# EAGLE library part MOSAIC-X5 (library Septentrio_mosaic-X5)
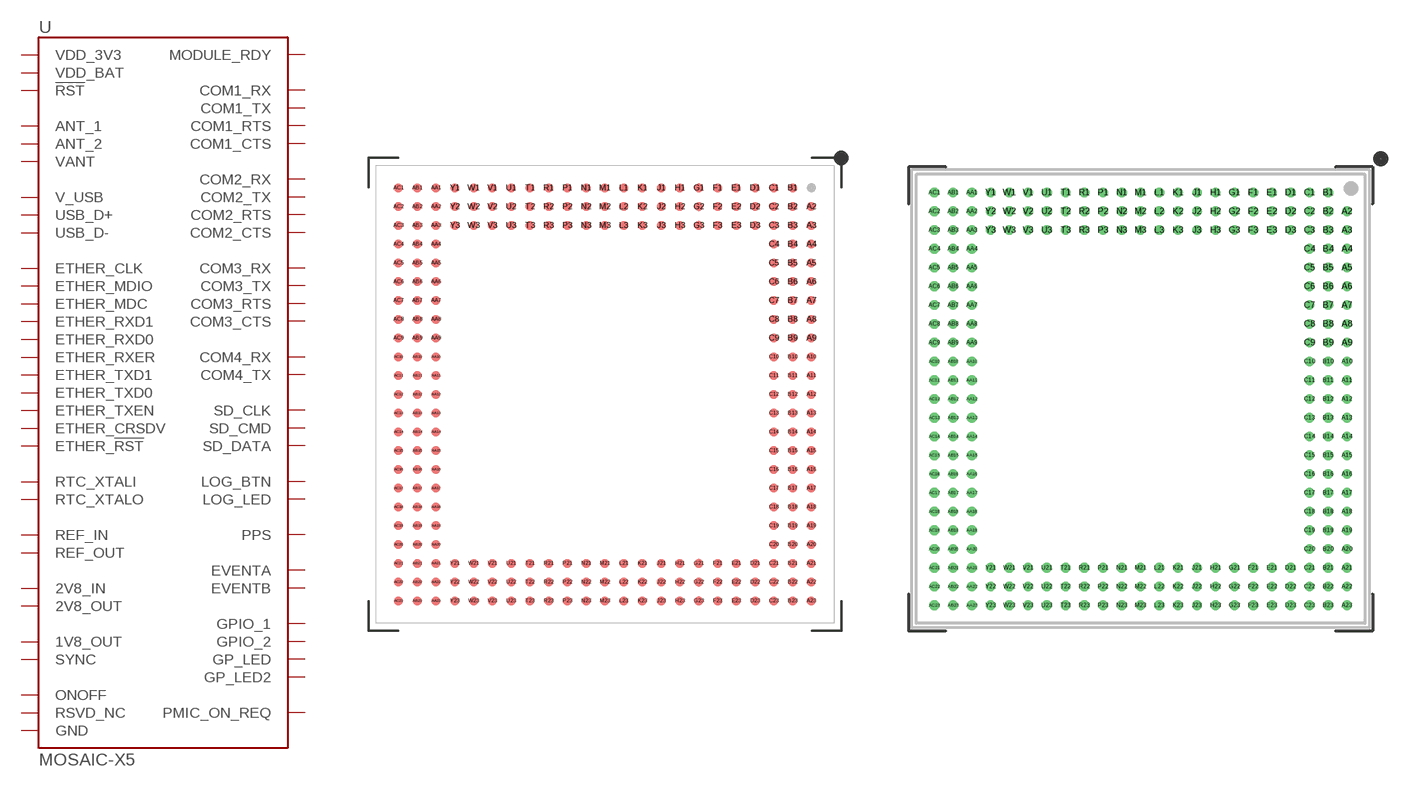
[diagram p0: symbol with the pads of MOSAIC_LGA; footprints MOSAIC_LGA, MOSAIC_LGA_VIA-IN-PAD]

Designator prefix -

## MOSAIC-X5X5 (PROD_ID: GPS-19395)  [MOSAIC_LGA]
A2  RTC_XTALO  out
A3  RTC_XTALI  in
A4  GND  pwr
A5  USB_D+
A6  USB_D-
A7  GND  pwr
A8  V_USB  in
A9  RSVD_NC  nc
A10  ONOFF  in
A11  !RST!  in
A12  MODULE_RDY  out
A13  RSVD_NC  nc
A14  GP_LED  out
A15  GND  pwr
A16  GND  pwr
A17  GND  pwr
A18  VDD_3V3  in
A19  VDD_3V3  in
A20  VDD_3V3  in
A21  GND  pwr
A22  GND  pwr
A23  GND  pwr
AA1  SD_CLK  out
AA2  ETHER_CLK  out
AA3  RSVD_NC  nc
AA4  GPIO_1  out
AA5  RSVD_NC  nc
AA6  RSVD_NC  nc
AA7  RSVD_NC  nc
AA8  RSVD_NC  nc
AA9  RSVD_NC  nc
AA10  RSVD_NC  nc
AA11  RSVD_NC  nc
AA12  RSVD_NC  nc
AA13  GND  pwr
AA14  GND  pwr
AA15  GND  pwr
AA16  GND  pwr
AA17  GND  pwr
AA18  GND  pwr
AA19  GND  pwr
AA20  GND  pwr
AA21  GND  pwr
AA22  GND  pwr
AA23  GND  pwr
AB1  SD_CMD  out
AB2  GND  pwr
AB3  GND  pwr
AB4  GND  pwr
AB5  GND  pwr
AB6  GND  pwr
AB7  GND  pwr
AB8  GND  pwr
AB9  RSVD_NC  nc
AB10  RSVD_NC  nc
AB11  RSVD_NC  nc
AB12  RSVD_NC  nc
AB13  GND  pwr
AB14  GND  pwr
AB15  GND  pwr
AB16  GND  pwr
AB17  GND  pwr
AB18  GND  pwr
AB19  GND  pwr
AB20  GND  pwr
AB21  GND  pwr
AB22  GND  pwr
AB23  GND  pwr
AC1  RSVD_NC  nc
AC2  RSVD_NC  nc
AC3  SYNC  in
AC4  1V8_OUT  out
AC5  RSVD_NC  nc
AC6  EVENTA  in
AC7  EVENTB  in
AC8  PPS  out
AC9  RSVD_NC  nc
AC10  RSVD_NC  nc
AC11  RSVD_NC  nc
AC12  RSVD_NC  nc
AC13  GND  pwr
AC14  RSVD_NC  nc
AC15  GND  pwr
AC16  REF_OUT  out
AC17  REF_IN  in
AC18  GND  pwr
AC19  GND  pwr
AC20  ANT_1  in
AC21  GND  pwr
AC22  GND  pwr
AC23  GND  pwr
B1  COM1_RX  in
B2  LOG_LED  out
B3  RSVD_NC  nc
B4  GND  pwr
B5  GND  pwr
B6  GND  pwr
B7  GND  pwr
B8  VDD_BAT  in
B9  RSVD_NC  nc
B10  RSVD_NC  nc
B11  RSVD_NC  nc
B12  RSVD_NC  nc
B13  GND  pwr
B14  RSVD_NC  nc
B15  RSVD_NC  nc
B16  PMIC_ON_REQ  out
B17  GND  pwr
B18  VDD_3V3  in
B19  VDD_3V3  in
B20  VDD_3V3  in
B21  GND  pwr
B22  RSVD_NC  nc
B23  RSVD_NC  nc
C1  COM1_RTS  out
C2  RSVD_NC  nc
C3  RSVD_NC  nc
C4  GND  pwr
C5  RSVD_NC  nc
C6  RSVD_NC  nc
C7  GND  pwr
C8  RSVD_NC  nc
C9  RSVD_NC  nc
C10  RSVD_NC  nc
C11  RSVD_NC  nc
C12  RSVD_NC  nc
C13  RSVD_NC  nc
C14  RSVD_NC  nc
C15  GND  pwr
C16  GND  pwr
C17  GND  pwr
C18  VDD_3V3  in
C19  VDD_3V3  in
C20  VDD_3V3  in
C21  RSVD_NC  nc
C22  RSVD_NC  nc
C23  GND  pwr
D1  COM1_TX  out
D2  GND  pwr
D3  COM4_RX  in
D21  GND  pwr
D22  GND  pwr
D23  GND  pwr
E1  COM1_CTS  in
E2  GND  pwr
E3  COM4_TX  out
E21  GND  pwr
E22  GND  pwr
E23  GND  pwr
F1  COM2_RX  in
F2  ETHER_!RST!  in
F3  RSVD_NC  nc
F21  GND  pwr
F22  GND  pwr
F23  GND  pwr
G1  COM2_RTS  out
G2  GND  pwr
G3  RSVD_NC  nc
G21  GND  pwr
G22  RSVD_NC  nc
G23  GND  pwr
H1  COM2_TX  out
H2  ETHER_TXD1  out
H3  RSVD_NC  nc
H21  GND  pwr
H22  GND  pwr
H23  GND  pwr
J1  COM2_CTS  in
J2  ETHER_TXD0  out
J3  RSVD_NC  nc
J21  GND  pwr
J22  GND  pwr
J23  GND  pwr
K1  COM3_RX  in
K2  GND  pwr
K3  LOG_BTN  in
K21  GND  pwr
K22  GND  pwr
K23  GND  pwr
L1  COM3_RTS  out
L2  ETHER_TXEN  out
L3  GPIO_2  out
L21  GND  pwr
L22  GND  pwr
L23  GND  pwr
M1  COM3_TX  out
M2  ETHER_RXER  in
M3  GP_LED2  out
M21  GND  pwr
M22  GND  pwr
M23  2V8_IN  in
N1  COM3_CTS  in
N2  ETHER_CRSDV  in
N3  RSVD_NC  nc
N21  GND  pwr
N22  GND  pwr
N23  2V8_OUT  out
P1  GND  pwr
P2  GND  pwr
P3  GND  pwr
P21  GND  pwr
P22  GND  pwr
P23  VANT  in
R1  RSVD_NC  nc
R2  ETHER_RXD0  in
R3  GND  pwr
R21  GND  pwr
R22  GND  pwr
R23  VANT  in
T1  RSVD_NC  nc
T2  ETHER_RXD1  in
T3  RSVD_NC  nc
T21  GND  pwr
T22  GND  pwr
T23  GND  pwr
U1  RSVD_NC  nc
U2  GND  pwr
U3  RSVD_NC  nc
U21  GND  pwr
U22  GND  pwr
U23  GND  pwr
V1  RSVD_NC  nc
V2  ETHER_MDC  out
V3  RSVD_NC  nc
V21  GND  pwr
V22  GND  pwr
V23  ANT_2  in
W1  RSVD_NC  nc
W2  ETHER_MDIO
W3  RSVD_NC  nc
W21  GND  pwr
W22  GND  pwr
W23  GND  pwr
Y1  SD_DATA
Y2  GND  pwr
Y3  RSVD_NC  nc
Y21  GND  pwr
Y22  GND  pwr
Y23  GND  pwr

## MOSAIC-X5X5_VIA-IN-PAD  [MOSAIC_LGA_VIA-IN-PAD]
Pads as for MOSAIC_LGA

## Footprint MOSAIC_LGA (pad centres in mm)
MOSAIC LGA - SMD
smd 0.6 x 0.6: A2 13.97,12.7; A3 13.97,11.43; A4 13.97,10.16; A5 13.97,8.89; A6 13.97,7.62; A7 13.97,6.35; A8 13.97,5.08; A9 13.97,3.81; A10 13.97,2.54; A11 13.97,1.27; A12 13.97,0; A13 13.97,-1.27; A14 13.97,-2.54; A15 13.97,-3.81; A16 13.97,-5.08; A17 13.97,-6.35; A18 13.97,-7.62; A19 13.97,-8.89; A20 13.97,-10.16; A21 13.97,-11.43; A22 13.97,-12.7; A23 13.97,-13.97; AA1 -11.43,13.97; AA2 -11.43,12.7; AA3 -11.43,11.43; AA4 -11.43,10.16; AA5 -11.43,8.89; AA6 -11.43,7.62; AA7 -11.43,6.35; AA8 -11.43,5.08; AA9 -11.43,3.81; AA10 -11.43,2.54; AA11 -11.43,1.27; AA12 -11.43,0; AA13 -11.43,-1.27; AA14 -11.43,-2.54; AA15 -11.43,-3.81; AA16 -11.43,-5.08; AA17 -11.43,-6.35; AA18 -11.43,-7.62; AA19 -11.43,-8.89; AA20 -11.43,-10.16; AA21 -11.43,-11.43; AA22 -11.43,-12.7; AA23 -11.43,-13.97; AB1 -12.7,13.97; AB2 -12.7,12.7; AB3 -12.7,11.43; AB4 -12.7,10.16; AB5 -12.7,8.89; AB6 -12.7,7.62; AB7 -12.7,6.35; AB8 -12.7,5.08; AB9 -12.7,3.81; AB10 -12.7,2.54; AB11 -12.7,1.27; AB12 -12.7,0; AB13 -12.7,-1.27; AB14 -12.7,-2.54; AB15 -12.7,-3.81; AB16 -12.7,-5.08; AB17 -12.7,-6.35; AB18 -12.7,-7.62; AB19 -12.7,-8.89; AB20 -12.7,-10.16; AB21 -12.7,-11.43; AB22 -12.7,-12.7; AB23 -12.7,-13.97; AC1 -13.97,13.97; AC2 -13.97,12.7; AC3 -13.97,11.43; AC4 -13.97,10.16; AC5 -13.97,8.89; AC6 -13.97,7.62; AC7 -13.97,6.35; AC8 -13.97,5.08; AC9 -13.97,3.81; AC10 -13.97,2.54; AC11 -13.97,1.27; AC12 -13.97,0; AC13 -13.97,-1.27; AC14 -13.97,-2.54; AC15 -13.97,-3.81; AC16 -13.97,-5.08; AC17 -13.97,-6.35; AC18 -13.97,-7.62; AC19 -13.97,-8.89; AC20 -13.97,-10.16; AC21 -13.97,-11.43; AC22 -13.97,-12.7; AC23 -13.97,-13.97; B1 12.7,13.97; B2 12.7,12.7; B3 12.7,11.43; B4 12.7,10.16; B5 12.7,8.89; B6 12.7,7.62; B7 12.7,6.35; B8 12.7,5.08; B9 12.7,3.81; B10 12.7,2.54; B11 12.7,1.27; B12 12.7,0; B13 12.7,-1.27; B14 12.7,-2.54; B15 12.7,-3.81; B16 12.7,-5.08; B17 12.7,-6.35; B18 12.7,-7.62; B19 12.7,-8.89; B20 12.7,-10.16; B21 12.7,-11.43; B22 12.7,-12.7; B23 12.7,-13.97; C1 11.43,13.97; C2 11.43,12.7; C3 11.43,11.43; C4 11.43,10.16; C5 11.43,8.89; C6 11.43,7.62; C7 11.43,6.35; C8 11.43,5.08; C9 11.43,3.81; C10 11.43,2.54; C11 11.43,1.27; C12 11.43,0; C13 11.43,-1.27; C14 11.43,-2.54; C15 11.43,-3.81; C16 11.43,-5.08; C17 11.43,-6.35; C18 11.43,-7.62; C19 11.43,-8.89; C20 11.43,-10.16; C21 11.43,-11.43; C22 11.43,-12.7; C23 11.43,-13.97; D1 10.16,13.97; D2 10.16,12.7; D3 10.16,11.43; D21 10.16,-11.43; D22 10.16,-12.7; D23 10.16,-13.97; E1 8.89,13.97; E2 8.89,12.7; E3 8.89,11.43; E21 8.89,-11.43; E22 8.89,-12.7; E23 8.89,-13.97; F1 7.62,13.97; F2 7.62,12.7; F3 7.62,11.43; F21 7.62,-11.43; F22 7.62,-12.7; F23 7.62,-13.97; G1 6.35,13.97; G2 6.35,12.7; G3 6.35,11.43; G21 6.35,-11.43; G22 6.35,-12.7; G23 6.35,-13.97; H1 5.08,13.97; H2 5.08,12.7; H3 5.08,11.43; H21 5.08,-11.43; H22 5.08,-12.7; H23 5.08,-13.97; J1 3.81,13.97; J2 3.81,12.7; J3 3.81,11.43; J21 3.81,-11.43; J22 3.81,-12.7; J23 3.81,-13.97; K1 2.54,13.97; K2 2.54,12.7; K3 2.54,11.43; K21 2.54,-11.43; K22 2.54,-12.7; K23 2.54,-13.97; L1 1.27,13.97; L2 1.27,12.7; L3 1.27,11.43; L21 1.27,-11.43; L22 1.27,-12.7; L23 1.27,-13.97; M1 0,13.97; M2 0,12.7; M3 0,11.43; M21 0,-11.43; M22 0,-12.7; M23 0,-13.97; N1 -1.27,13.97; N2 -1.27,12.7; N3 -1.27,11.43; N21 -1.27,-11.43; N22 -1.27,-12.7; N23 -1.27,-13.97; P1 -2.54,13.97; P2 -2.54,12.7; P3 -2.54,11.43; P21 -2.54,-11.43; P22 -2.54,-12.7; P23 -2.54,-13.97; R1 -3.81,13.97; R2 -3.81,12.7; R3 -3.81,11.43; R21 -3.81,-11.43; R22 -3.81,-12.7; R23 -3.81,-13.97; T1 -5.08,13.97; T2 -5.08,12.7; T3 -5.08,11.43; T21 -5.08,-11.43; T22 -5.08,-12.7; T23 -5.08,-13.97; U1 -6.35,13.97; U2 -6.35,12.7; U3 -6.35,11.43; U21 -6.35,-11.43; U22 -6.35,-12.7; U23 -6.35,-13.97; V1 -7.62,13.97; V2 -7.62,12.7; V3 -7.62,11.43; V21 -7.62,-11.43; V22 -7.62,-12.7; V23 -7.62,-13.97; W1 -8.89,13.97; W2 -8.89,12.7; W3 -8.89,11.43; W21 -8.89,-11.43; W22 -8.89,-12.7; W23 -8.89,-13.97; Y1 -10.16,13.97; Y2 -10.16,12.7; Y3 -10.16,11.43; Y21 -10.16,-11.43; Y22 -10.16,-12.7; Y23 -10.16,-13.97

## Footprint MOSAIC_LGA_VIA-IN-PAD (pad centres in mm)
MOSAIC LGA - via-in-pad
drill 0.15 pad 0.6: A2 13.97,12.7; A3 13.97,11.43; A4 13.97,10.16; A5 13.97,8.89; A6 13.97,7.62; A7 13.97,6.35; A8 13.97,5.08; A9 13.97,3.81; A10 13.97,2.54; A11 13.97,1.27; A12 13.97,0; A13 13.97,-1.27; A14 13.97,-2.54; A15 13.97,-3.81; A16 13.97,-5.08; A17 13.97,-6.35; A18 13.97,-7.62; A19 13.97,-8.89; A20 13.97,-10.16; A21 13.97,-11.43; A22 13.97,-12.7; A23 13.97,-13.97; AA1 -11.43,13.97; AA2 -11.43,12.7; AA3 -11.43,11.43; AA4 -11.43,10.16; AA5 -11.43,8.89; AA6 -11.43,7.62; AA7 -11.43,6.35; AA8 -11.43,5.08; AA9 -11.43,3.81; AA10 -11.43,2.54; AA11 -11.43,1.27; AA12 -11.43,0; AA13 -11.43,-1.27; AA14 -11.43,-2.54; AA15 -11.43,-3.81; AA16 -11.43,-5.08; AA17 -11.43,-6.35; AA18 -11.43,-7.62; AA19 -11.43,-8.89; AA20 -11.43,-10.16; AA21 -11.43,-11.43; AA22 -11.43,-12.7; AA23 -11.43,-13.97; AB1 -12.7,13.97; AB2 -12.7,12.7; AB3 -12.7,11.43; AB4 -12.7,10.16; AB5 -12.7,8.89; AB6 -12.7,7.62; AB7 -12.7,6.35; AB8 -12.7,5.08; AB9 -12.7,3.81; AB10 -12.7,2.54; AB11 -12.7,1.27; AB12 -12.7,0; AB13 -12.7,-1.27; AB14 -12.7,-2.54; AB15 -12.7,-3.81; AB16 -12.7,-5.08; AB17 -12.7,-6.35; AB18 -12.7,-7.62; AB19 -12.7,-8.89; AB20 -12.7,-10.16; AB21 -12.7,-11.43; AB22 -12.7,-12.7; AB23 -12.7,-13.97; AC1 -13.97,13.97; AC2 -13.97,12.7; AC3 -13.97,11.43; AC4 -13.97,10.16; AC5 -13.97,8.89; AC6 -13.97,7.62; AC7 -13.97,6.35; AC8 -13.97,5.08; AC9 -13.97,3.81; AC10 -13.97,2.54; AC11 -13.97,1.27; AC12 -13.97,0; AC13 -13.97,-1.27; AC14 -13.97,-2.54; AC15 -13.97,-3.81; AC16 -13.97,-5.08; AC17 -13.97,-6.35; AC18 -13.97,-7.62; AC19 -13.97,-8.89; AC20 -13.97,-10.16; AC21 -13.97,-11.43; AC22 -13.97,-12.7; AC23 -13.97,-13.97; B1 12.7,13.97; B2 12.7,12.7; B3 12.7,11.43; B4 12.7,10.16; B5 12.7,8.89; B6 12.7,7.62; B7 12.7,6.35; B8 12.7,5.08; B9 12.7,3.81; B10 12.7,2.54; B11 12.7,1.27; B12 12.7,0; B13 12.7,-1.27; B14 12.7,-2.54; B15 12.7,-3.81; B16 12.7,-5.08; B17 12.7,-6.35; B18 12.7,-7.62; B19 12.7,-8.89; B20 12.7,-10.16; B21 12.7,-11.43; B22 12.7,-12.7; B23 12.7,-13.97; C1 11.43,13.97; C2 11.43,12.7; C3 11.43,11.43; C4 11.43,10.16; C5 11.43,8.89; C6 11.43,7.62; C7 11.43,6.35; C8 11.43,5.08; C9 11.43,3.81; C10 11.43,2.54; C11 11.43,1.27; C12 11.43,0; C13 11.43,-1.27; C14 11.43,-2.54; C15 11.43,-3.81; C16 11.43,-5.08; C17 11.43,-6.35; C18 11.43,-7.62; C19 11.43,-8.89; C20 11.43,-10.16; C21 11.43,-11.43; C22 11.43,-12.7; C23 11.43,-13.97; D1 10.16,13.97; D2 10.16,12.7; D3 10.16,11.43; D21 10.16,-11.43; D22 10.16,-12.7; D23 10.16,-13.97; E1 8.89,13.97; E2 8.89,12.7; E3 8.89,11.43; E21 8.89,-11.43; E22 8.89,-12.7; E23 8.89,-13.97; F1 7.62,13.97; F2 7.62,12.7; F3 7.62,11.43; F21 7.62,-11.43; F22 7.62,-12.7; F23 7.62,-13.97; G1 6.35,13.97; G2 6.35,12.7; G3 6.35,11.43; G21 6.35,-11.43; G22 6.35,-12.7; G23 6.35,-13.97; H1 5.08,13.97; H2 5.08,12.7; H3 5.08,11.43; H21 5.08,-11.43; H22 5.08,-12.7; H23 5.08,-13.97; J1 3.81,13.97; J2 3.81,12.7; J3 3.81,11.43; J21 3.81,-11.43; J22 3.81,-12.7; J23 3.81,-13.97; K1 2.54,13.97; K2 2.54,12.7; K3 2.54,11.43; K21 2.54,-11.43; K22 2.54,-12.7; K23 2.54,-13.97; L1 1.27,13.97; L2 1.27,12.7; L3 1.27,11.43; L21 1.27,-11.43; L22 1.27,-12.7; L23 1.27,-13.97; M1 0,13.97; M2 0,12.7; M3 0,11.43; M21 0,-11.43; M22 0,-12.7; M23 0,-13.97; N1 -1.27,13.97; N2 -1.27,12.7; N3 -1.27,11.43; N21 -1.27,-11.43; N22 -1.27,-12.7; N23 -1.27,-13.97; P1 -2.54,13.97; P2 -2.54,12.7; P3 -2.54,11.43; P21 -2.54,-11.43; P22 -2.54,-12.7; P23 -2.54,-13.97; R1 -3.81,13.97; R2 -3.81,12.7; R3 -3.81,11.43; R21 -3.81,-11.43; R22 -3.81,-12.7; R23 -3.81,-13.97; T1 -5.08,13.97; T2 -5.08,12.7; T3 -5.08,11.43; T21 -5.08,-11.43; T22 -5.08,-12.7; T23 -5.08,-13.97; U1 -6.35,13.97; U2 -6.35,12.7; U3 -6.35,11.43; U21 -6.35,-11.43; U22 -6.35,-12.7; U23 -6.35,-13.97; V1 -7.62,13.97; V2 -7.62,12.7; V3 -7.62,11.43; V21 -7.62,-11.43; V22 -7.62,-12.7; V23 -7.62,-13.97; W1 -8.89,13.97; W2 -8.89,12.7; W3 -8.89,11.43; W21 -8.89,-11.43; W22 -8.89,-12.7; W23 -8.89,-13.97; Y1 -10.16,13.97; Y2 -10.16,12.7; Y3 -10.16,11.43; Y21 -10.16,-11.43; Y22 -10.16,-12.7; Y23 -10.16,-13.97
